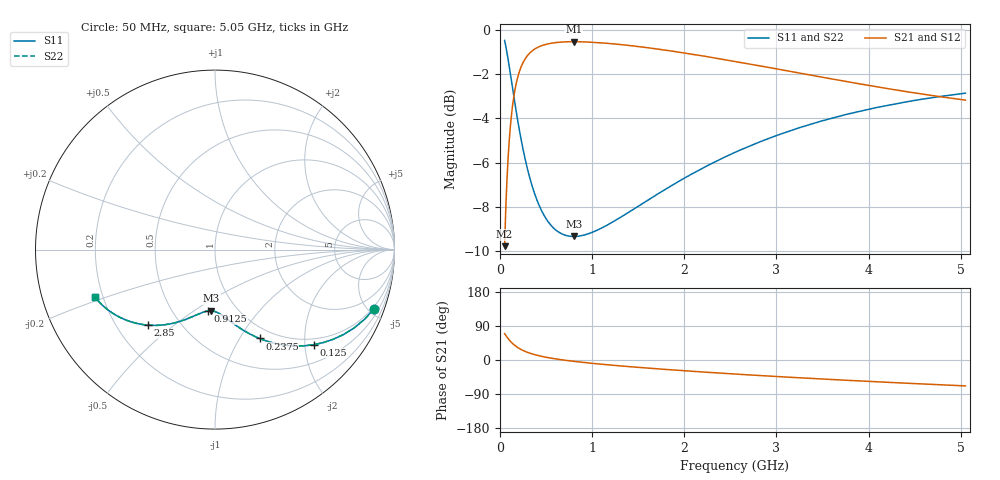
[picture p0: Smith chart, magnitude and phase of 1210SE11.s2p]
! AVX Thin Film Operation		Date: August 2001
! Description: Accu-P® Series, Thin Film, SMD, RF Capacitor
! Part Number: 12101J110FBT
! 50 MHz  -  5.05 GHz
! Serial Measurements
# mhz S db R 50
!	S11		S21		S12		S22
!	dB	Phase	dB	Phase	dB	Phase	dB	Phase
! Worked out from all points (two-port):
!   401 points, 50 MHz to 5.05 GHz, reference 50 ohm
!   highest |S21| = -0.54 dB at 800 MHz (marker M1); lowest = -9.8 dB at 50 MHz (marker M2)
!   |S21| within 3 dB of the highest: 133.2 MHz to end of sweep
!   lowest |S11| = -9.3 dB at 800 MHz (marker M3), VSWR 2.04, Z = 38.1 - j29.4 ohm
!   |S11| at or under -10 dB: nowhere
!   |S22| runs from -9.3 to -0.5 dB; largest |S21 - S12| = 0
!   S11 on the Smith chart (normalised r, x): 50 MHz: 0.86, -5.41; 125 MHz: 0.86, -2.20; 237.5 MHz: 0.86, -1.22; 912.5 MHz: 0.74, -0.57; 2.85 GHz: 0.33, -0.41; 5.05 GHz: 0.17, -0.19
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50  -0.48 -20.4  -9.77 69.6  -9.77 69.6  -0.48 -20.4
75  -1.01 -29.4  -6.82 60.6  -6.82 60.6  -1.01 -29.4
100  -1.65 -37.1  -5.02 52.9  -5.02 52.9  -1.65 -37.1
125  -2.32 -43.8  -3.83 46.2  -3.83 46.2  -2.32 -43.8
175  -3.66 -54.2  -2.44 35.8  -2.44 35.8  -3.66 -54.2
200  -4.29 -58.3  -2.03 31.7  -2.03 31.7  -4.29 -58.3
237.5  -5.13 -63.4  -1.59 26.6  -1.59 26.6  -5.13 -63.4
275  -5.88 -67.6  -1.30 22.4  -1.30 22.4  -5.88 -67.6
325  -6.71 -72.1  -1.04 17.9  -1.04 17.9  -6.71 -72.1
437.5  -8.05 -79.6  -0.74 10.4  -0.74 10.4  -8.05 -79.6
600  -9.02 -86.9  -0.58 3.0  -0.58 3.0  -9.02 -86.9
800  -9.33 -93.5  -0.54 -3.5  -0.54 -3.5  -9.33 -93.5
887.5  -9.29 -95.9  -0.55 -5.9  -0.55 -5.9  -9.29 -95.9
912.5  -9.27 -96.5  -0.55 -6.6  -0.55 -6.6  -9.27 -96.5
1275  -8.55 -104.9  -0.66 -14.9  -0.66 -14.9  -8.55 -104.9
1725  -7.38 -113.6  -0.88 -23.6  -0.88 -23.6  -7.38 -113.6
2125  -6.41 -120.4  -1.13 -30.4  -1.13 -30.4  -6.41 -120.4
2550  -5.53 -127.1  -1.43 -37.1  -1.43 -37.1  -5.54 -127.1
2850  -5.01 -131.4  -1.65 -41.5  -1.65 -41.5  -5.01 -131.4
3387.5  -4.24 -138.8  -2.06 -48.8  -2.06 -48.8  -4.24 -138.8
4225  -3.40 -149.1  -2.67 -59.1  -2.67 -59.1  -3.40 -149.1
5050  -2.87 -158.3  -3.18 -68.4  -3.18 -68.4  -2.87 -158.3
